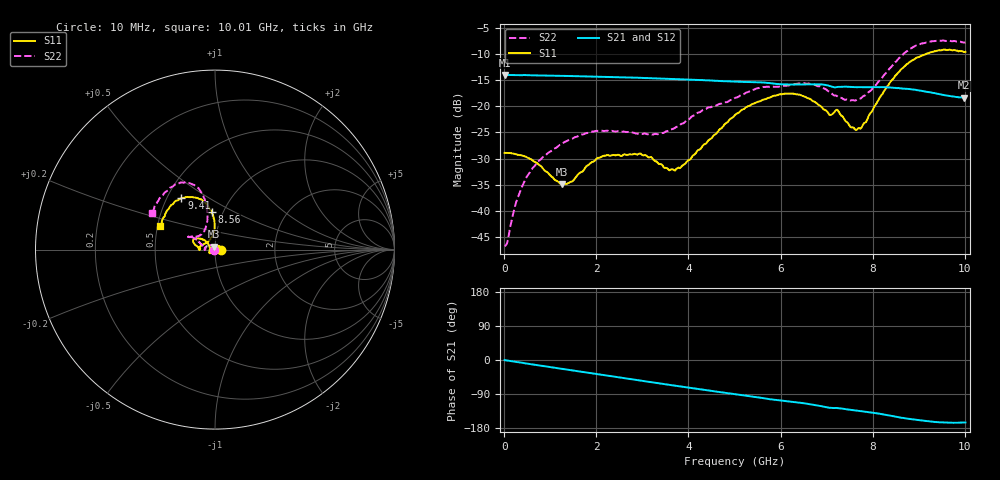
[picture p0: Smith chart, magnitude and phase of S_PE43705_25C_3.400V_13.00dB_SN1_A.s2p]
! Device ID: PE43705
! Serial: 1
! Insertion: A
! Impedance: 50 ohm
! Temp: 25C
! VDD: 3.400V
! Attenuation Step: 13.00dB
#  Hz  S  RI  R  50
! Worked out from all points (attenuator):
!   401 points, 10 MHz to 10.01 GHz, reference 50 ohm
!   highest |S21| = -13.98 dB at 10 MHz (marker M1); lowest = -18.3 dB at 9.985 GHz (marker M2)
!   lowest |S11| = -34.9 dB at 1.26 GHz (marker M3), VSWR 1.04, Z = 49.5 + j1.7 ohm
!   |S11| at or under -10 dB: start of sweep to 9.159 GHz
!   |S22| runs from -46.8 to -7.4 dB; largest |S21 - S12| = 0.0019
!   S11 on the Smith chart (normalised r, x): 10 MHz: 1.07, +0.00; 8.56 GHz: 0.88, +0.39; 9.41 GHz: 0.59, +0.38; 10.01 GHz: 0.52, +0.15
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1e7  0.0358 0.000219  0.1999 -0.000935  0.2002 -0.000846  -0.00457 0.00043
2.85e8  0.033 0.00981  0.1976 -0.019  0.1977 -0.019  -0.00551 0.0118
4.85e8  0.0283 0.0165  0.1958 -0.0323  0.1959 -0.0321  -0.00934 0.0188
7.85e8  0.0164 0.0214  0.1907 -0.0507  0.1907 -0.0506  -0.019 0.0242
1.26e9  -0.00519 0.0172  0.1789 -0.0784  0.1791 -0.0782  -0.0374 0.0227
1.685e9  -0.0228 0.00579  0.1653 -0.1008  0.1653 -0.1007  -0.0517 0.0147
2.21e9  -0.032 -0.0115  0.1445 -0.1253  0.1446 -0.1252  -0.0583 0.00301
2.96e9  -0.0288 -0.0206  0.1085 -0.1525  0.1088 -0.1523  -0.0545 0.00273
3.36e9  -0.0237 -0.0151  0.0877 -0.1622  0.0879 -0.162  -0.054 0.00626
3.86e9  -0.0265 0.00506  0.0607 -0.1705  0.0609 -0.1704  -0.0653 0.0198
5.01e9  -0.0621 0.0546  2.72e-05 -0.1723  0.000184 -0.1723  -0.1061 0.0566
5.985e9  -0.1162 0.0589  -0.0461 -0.1561  -0.0453 -0.1564  -0.1359 0.0735
6.685e9  -0.1105 0.0264  -0.0752 -0.1436  -0.0751 -0.1437  -0.1447 0.0708
7.06e9  -0.0826 0.00605  -0.0919 -0.1264  -0.0916 -0.1268  -0.1159 0.074
7.235e9  -0.0916 0.0116  -0.0919 -0.1225  -0.0916 -0.1223  -0.1007 0.0725
7.685e9  -0.0352 0.0509  -0.1058 -0.11  -0.106 -0.11  -0.0641 0.0984
8.36e9  -0.004 0.1655  -0.1264 -0.0837  -0.1256 -0.0841  -0.0453 0.2239
8.56e9  -0.0189 0.211  -0.1312 -0.0724  -0.1297 -0.073  -0.0566 0.2805
8.935e9  -0.074 0.279  -0.1329 -0.0546  -0.1327 -0.0532  -0.1196 0.3618
9.41e9  -0.1871 0.2864  -0.1268 -0.036  -0.1264 -0.036  -0.2198 0.3647
9.985e9  -0.2985 0.1406  -0.117 -0.0315  -0.117 -0.032  -0.3454 0.2141
1.001e10  -0.3049 0.1312  -0.1176 -0.0319  -0.1177 -0.0323  -0.3531 0.2033
